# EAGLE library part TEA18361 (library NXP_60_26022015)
GreenChip SMPS control IC The TEA18361T is a controller IC for low-cost Switched Mode Power Supplies (SMPS). It is intended for flyback topologies. The built-in green functions provide high efficiency at all power levels. At high power levels the flyback operates in Quasi-Resonant (QR) mode. At lower power levels, the controller switches to Frequency Reduction (FR) or Discontinuous Conduction Mode (DCM) and limits the peak current to approximately 25 % of the maximum peak current. Valley switching is used in all operating modes. At low power levels, when the flyback switching frequency drops below 25 kHz, the flyback converter switches to burst mode. A special burst mode has been integrated which reduces the opto current to a minimum level, ensuring high efficiency at low power and excellent no load power performance. As the switching frequency in this mode has a minimum value of 25 kHz while the burst frequency is below 800 Hz, the frequencies are outside the audible range. During the non-switching phase of the burst mode, the internal IC supply current is minimized for further efficiency optimization. The TEA18361T includes an accurate OverPower Protection (OPP). The OPP enables the controller to operate in overpower situations for a limited amount of time. If the output is shorted, the system switches to low-power mode where the output power is limited to a lower level. The TEA18361T is manufactured in a high-voltage Silicon-On-Insulator (SOI) process. The SOI process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
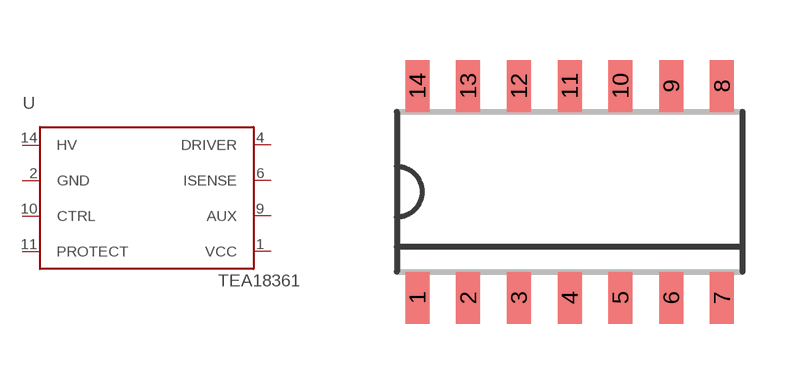
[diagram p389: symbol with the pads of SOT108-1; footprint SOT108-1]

Designator prefix U

## TEA18361T  [SOT108-1]
1  VCC
2  GND
4  DRIVER
6  ISENSE
9  AUX
10  CTRL
11  PROTECT
14  HV

## Footprint SOT108-1 (pad centres in mm)
SOT108-1 SO14: plastic small outline package; 14 leads; body width 3.9 mm; body thickness 1.47 mm JEDEC: MS-012 IEC: --
smd 0.6 x 1.3: 1 -3.81,-2.65; 2 -2.54,-2.65; 3 -1.27,-2.65; 4 0,-2.65; 5 1.27,-2.65; 6 2.54,-2.65; 7 3.81,-2.65; 8 3.81,2.65; 9 2.54,2.65; 10 1.27,2.65; 11 0,2.65; 12 -1.27,2.65; 13 -2.54,2.65; 14 -3.81,2.65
